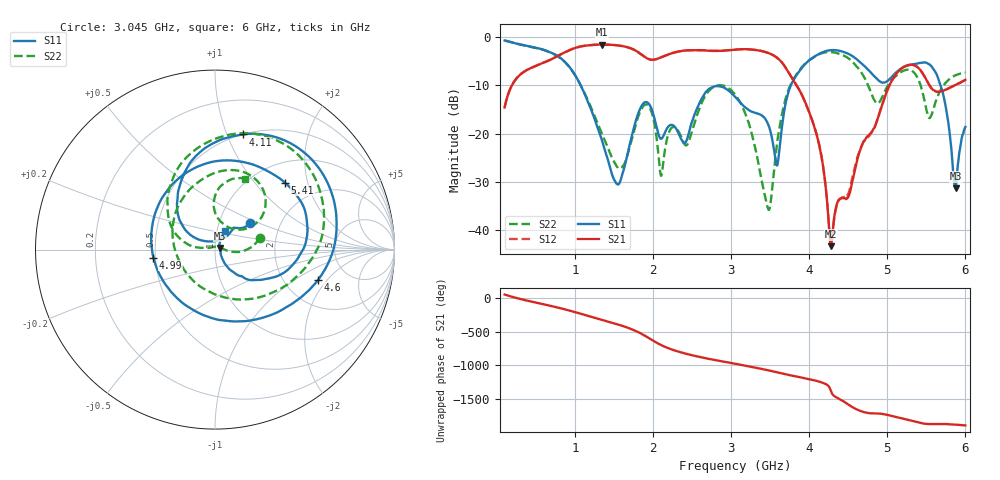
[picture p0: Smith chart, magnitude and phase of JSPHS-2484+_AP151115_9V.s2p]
!Mini-Circuits Laboratory
!S-Parameters
!Run/Lot/Date Code:MF33450/NA/1551
!Fixture/SN/Due: 90-4-20-21/70546/03/17/16
!Connection:PORT<IN> - pin<1>; PORT<OUT> - pin<7>;PORT<BIAS> - pin<4>;
!Tested With:PORT EXTENTION
!Network Analyzer:AG E5071C/74883/05/12/16
!Created: 01-07-2016 at 14:10:27
!MODEL: JSPHS-2484+
!S/N: V=9V
# MHZ S DB R 50
!Frequency  S11 dB  S11 DEG  S21 dB  S21 DEG  S12 dB  S12 DEG  S22 dB  S22 DEG
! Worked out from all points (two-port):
!   1181 points, 100 MHz to 6 GHz, reference 50 ohm
!   highest |S21| = -1.51 dB at 1.35 GHz (marker M1); lowest = -43.4 dB at 4.275 GHz (marker M2)
!   |S21| within 3 dB of the highest: 706.7 MHz to 1.941 GHz (1.234 GHz wide, 93.2 % of centre); 2.048 GHz to 3.607 GHz (1.559 GHz wide, 55.1 % of centre)
!   lowest |S11| = -31.4 dB at 5.875 GHz (marker M3), VSWR 1.06, Z = 52.6 + j0.914 ohm
!   |S11| at or under -10 dB: 1.074 GHz to 3.765 GHz (2.691 GHz wide, 111 % of centre); 5.683 GHz to end of sweep
!   |S22| runs from -35.9 to -0.7 dB; largest |S21 - S12| = 0.0038
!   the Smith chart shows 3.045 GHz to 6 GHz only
!   S11 on the Smith chart (normalised r, x): 3.045 GHz: 1.40, +0.44; 4.11 GHz: 0.50, +1.14; 4.6 GHz: 3.07, -1.61; 4.99 GHz: 0.49, -0.05; 5.41 GHz: 1.39, +1.46; 6 GHz: 1.09, +0.23
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100  -0.67 -38.5  -14.58 51.2  -14.57 51.1  -0.66 -38.5
530  -2.28 -163.8  -5.73 -75.7  -5.73 -75.7  -2.32 -167.1
815  -4.30 122.7  -3.58 -151.5  -3.57 -151.6  -4.36 118.2
1085  -10.38 38.7  -1.87 122.8  -1.87 122.8  -10.31 33.9
1350  -21.62 -48.7  -1.51 36.1  -1.51 36.1  -20.20 -66.1
1685  -23.50 149.0  -2.13 -85.0  -2.12 -85.0  -23.83 177.1
1865  -13.98 77.4  -3.75 -179.5  -3.75 -179.6  -14.55 90.1
2070  -20.15 20.7  -4.38 41.5  -4.38 41.5  -24.44 -0.7
2390  -21.93 54.1  -2.78 -97.2  -2.78 -97.2  -21.75 47.5
2675  -11.40 77.3  -2.75 -174.6  -2.74 -174.6  -11.98 77.0
3045  -12.27 37.3  -2.58 105.7  -2.58 105.7  -11.79 15.2
3050  -12.36 37.1  -2.57 104.7  -2.57 104.6  -11.90 14.4
3480  -18.31 48.0  -3.29 5.5  -3.28 5.5  -35.85 93.5
4035  -4.36 88.5  -17.08 -134.0  -17.06 -133.2  -4.37 93.0
4110  -3.61 76.5  -21.15 -155.2  -21.05 -155.3  -3.66 79.9
4275  -2.68 47.6  -43.40 68.9  -43.21 70.5  -3.06 50.1
4600  -4.45 -16.3  -26.59 151.1  -26.10 149.6  -5.90 -12.6
4990  -9.22 -172.6  -11.43 67.6  -11.45 67.4  -10.54 138.4
5020  -8.84 170.1  -10.25 59.8  -10.25 59.6  -9.72 126.4
5410  -5.36 43.7  -6.55 -51.0  -6.56 -51.1  -9.24 37.6
5875  -31.40 18.8  -9.91 -79.3  -9.89 -79.3  -7.88 76.6
6000  -18.64 61.8  -8.84 -91.7  -8.86 -91.7  -7.37 67.3
